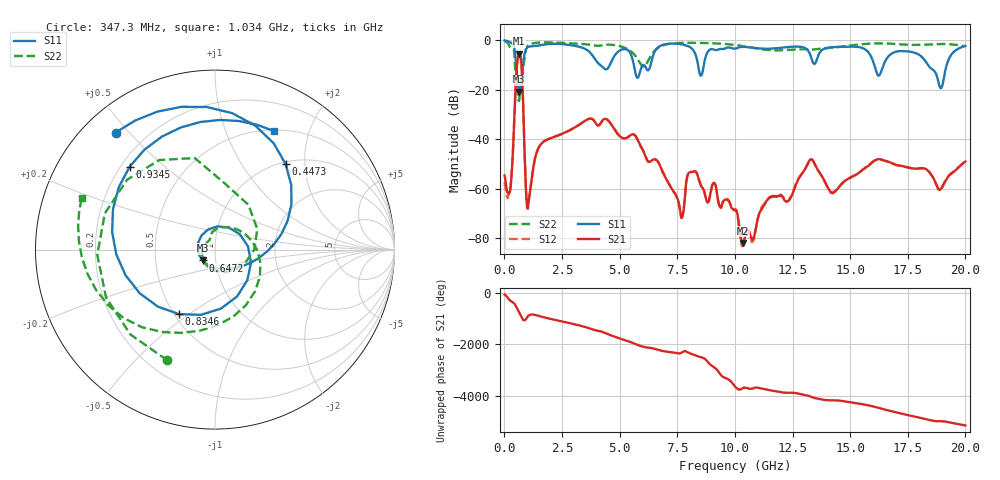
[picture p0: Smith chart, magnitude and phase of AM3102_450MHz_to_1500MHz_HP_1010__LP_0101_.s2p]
!Agilent Technologies,E8364B,MY43040894,A.07.50.67
!Agilent E8364B: A.07.50.67
!Date: Thursday, January 11, 2018 06:11:09
!Correction: S11(Full 2 Port(1,2))
!S21(Full 2 Port(1,2))
!S12(Full 2 Port(1,2))
!S22(Full 2 Port(1,2))
!S2P File: Measurements: S11, S21, S12, S22:
# Hz S  dB  R 50
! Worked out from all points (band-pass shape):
!   1601 points, 10 MHz to 20 GHz, reference 50 ohm
!   highest |S21| = -5.39 dB at 634.7 MHz (marker M1); lowest = -81.9 dB at 10.34 GHz (marker M2)
!   |S21| within 3 dB of the highest: 562.5 MHz to 726.8 MHz (164.3 MHz wide, 25.5 % of centre)
!   lowest |S11| = -20.8 dB at 647.2 MHz (marker M3), VSWR 1.20, Z = 43.3 - j5.28 ohm
!   |S11| at or under -10 dB: 4.158 GHz to 4.573 GHz (414.8 MHz wide, 9.5 % of centre); 5.616 GHz to 6.011 GHz (395.3 MHz wide, 6.8 % of centre); 18.38 GHz to 19.19 GHz (811.2 MHz wide, 4.32 % of centre)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
!   |S22| runs from -24.5 to -0.4 dB; largest |S21 - S12| = 0.0032
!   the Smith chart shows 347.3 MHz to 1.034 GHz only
!   S11 on the Smith chart (normalised r, x): 347.3 MHz: 0.09, +0.46; 447.3 MHz: 1.04, +1.60; 647.2 MHz: 0.87, -0.11; 834.6 MHz: 0.53, -0.46; 934.5 MHz: 0.23, +0.39; 1.034 GHz: 0.51, +1.49
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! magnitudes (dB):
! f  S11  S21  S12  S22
! 10 MHz  -0.1  -54.7  -57.5  -0.4
! 209.9 MHz  -0.6  -61.6  -62.1  -2.2
! 347.3 MHz  -1.4  -49.3  -49.1  -3.5
! 447.3 MHz  -4.2  -27.0  -26.9  -8.6
! 634.7 MHz  -20.6  -5.4  -5.4  -24.5
! 647.2 MHz  -20.8  -5.4  -5.4  -24.2
! 834.6 MHz  -7.7  -32.7  -33.0  -9.8
! 934.5 MHz  -3.6  -60.0  -60.2  -3.9
! 1.034 GHz  -2.6  -66.7  -66.9  -2.0
! 1.559 GHz  -2.0  -42.3  -42.3  -0.9
! 3.346 GHz  -2.9  -33.5  -33.5  -1.5
! 5.782 GHz  -15.2  -40.2  -40.2  -7.6
! 6.682 GHz  -2.8  -49.4  -49.4  -2.9
! 7.681 GHz  -1.6  -71.8  -71.4  -1.0
! 8.206 GHz  -4.1  -53.1  -53.2  -1.0
! 10.01 GHz  -3.4  -68.6  -68.5  -1.9
! 10.34 GHz  -2.7  -81.9  -82.9  -2.3
! 13.34 GHz  -7.8  -48.2  -48.2  -3.8
! 14.24 GHz  -2.8  -61.9  -61.5  -3.0
! 16.68 GHz  -6.3  -49.2  -49.2  -1.3
! 18.94 GHz  -19.4  -60.1  -60.2  -1.5
! 20 GHz  -2.3  -49.0  -49.0  -2.3
